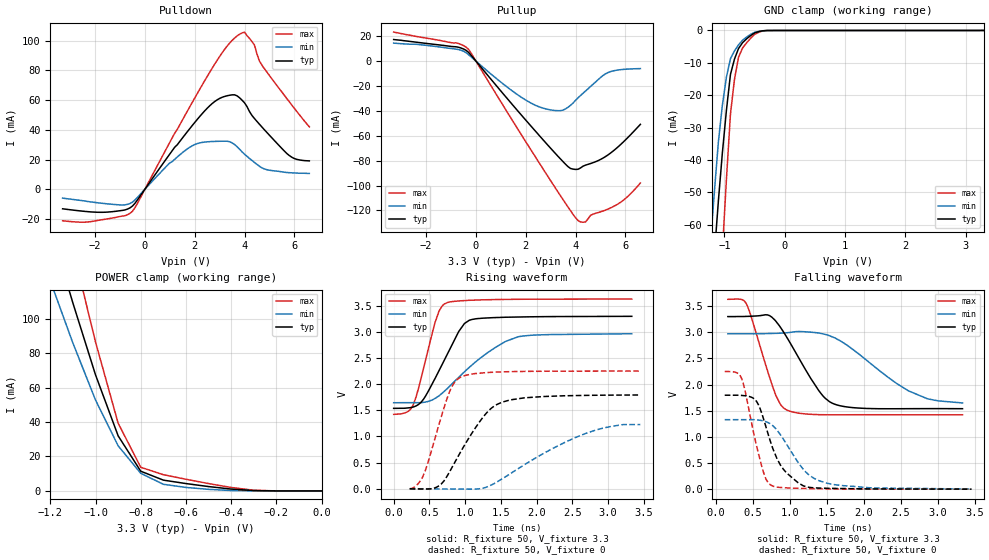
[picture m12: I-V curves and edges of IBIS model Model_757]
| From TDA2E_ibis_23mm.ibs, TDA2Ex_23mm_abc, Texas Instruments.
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| Model based on original model for BC1833DV40DCPBFBP1811_SSCEV
|   Sub model BC40D_V_10P_SC1_3P3
[model]   Model_757
|[Description]  [3.3V-I/O-X-40C CLASS MODE SLOW MODE, IND, 10 PERCENT%]
|   40C CLASS MODE SLOW MODE, ,IND,10 PERCENT%
|[Input Load]
|[Output Drive] 40C CLASS MODE SLOW MODE
|Voltage   3.3V
|Mode   I/O
Model_type   I/O
Polarity   Non-Inverting
Enable   Active-Low
Vinl =  0.8V
Vinh =  2V
Cref =  15pF
Rref =  100.0000M
Vref =  0V
Vmeas =  1.65
C_comp   2.155p   1.84p   2.47p
[Model Spec]
Vinl   0.8V   0.8V   0.8V
Vinh   2V   2V   2V
D_overshoot_ampl_h 0.66 0.66 0.66
D_overshoot_ampl_l 0.66 0.66 0.66
D_overshoot_area_h 0.33n 0.33n 0.33n
D_overshoot_area_l 0.33n 0.33n 0.33n
D_overshoot_high 3.96 3.96 3.96
D_overshoot_low -0.66 -0.66 -0.66
D_overshoot_time 1n 1n 1n
S_overshoot_high 3.3 3.3 3.3
S_overshoot_low 0 0 0
[Temperature Range]   25   125   -40
[Voltage Range]   3.3   2.97   3.63
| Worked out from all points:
|   slope of the pulldown table from 0 to 0.495 V, typ, clamps not added: 41.8 ohm
|   slope of the pullup table from 0 to 0.495 V, typ, clamps not added: 41.4 ohm
|   GND clamp passes 1 mA (typ) near -0.52 V on its own axis
|   POWER clamp passes 1 mA (typ) near -0.39 V on its own axis
|   rising waveform, R_fixture 50, V_fixture 3.3: 20-80 % time 393ps typ, 678ps min, 244ps max; typ from 1.54 V to 3.3 V
|   rising waveform, R_fixture 50, V_fixture 0: 20-80 % time 493ps typ, 965ps min, 299ps max; typ from -0.001 V to 1.79 V
|   falling waveform, R_fixture 50, V_fixture 3.3: 20-80 % time 448ps typ, 747ps min, 291ps max; typ from 3.3 V to 1.54 V
|   falling waveform, R_fixture 50, V_fixture 0: 20-80 % time 302ps typ, 402ps min, 211ps max; typ from 1.8 V to 0.001 V
[POWER_clamp]
-3.3V     1.165A     1.155A     1.459A
-1.2V     153.4mA    122mA      196.7mA
-1.167V   138.6mA    109.9mA    177.9mA
-1.1V     109.1mA    85.82mA    140.3mA
-1.067V   95.17mA    74.8mA     122.3mA
-1.033V   81.28mA    63.79mA    104.4mA
-900mV    31.99mA    26.19mA    39.32mA
-800mV    11.44mA    10.22mA    13.73mA
-700mV    6.266mA    3.856mA    9.428mA
-600mV    4.272mA    2.023mA    6.777mA
-300mV    202.9uA    25.56uA    396.8uA
0V        3.057uA    1.011uA    8.442uA
[Pulldown]
-3.3V     -13.12mA   -5.96mA    -21.19mA
-1.6V     -15.42mA   -9.62mA    -20.15mA
-500mV    -11.32mA   -8.666mA   -14.78mA
1V        23.71mA    17.75mA    31.58mA
2V        44.93mA    30.08mA    61.37mA
3V        61.12mA    32.31mA    89.33mA
3.6V      63.57mA    30.09mA    101.8mA
3.9V      59.97mA    25.19mA    105.2mA
4.4V      47.59mA    18.06mA    96.94mA
4.7V      41.87mA    14.42mA    83.43mA
5.7V      24.04mA    11.3mA     61mA
6.6V      19.1mA     10.7mA     42mA
[Pullup]
-3.3V     17.3mA     14.4mA     23.3mA
-300mV    7.112mA    5.275mA    9.555mA
1.4V      -33.47mA   -23.08mA   -45.6mA
2.5V      -58.82mA   -36.46mA   -80.5mA
3.4V      -78.75mA   -39.82mA   -108.4mA
3.8V      -86.3mA    -35.51mA   -120.3mA
4.1V      -86.92mA   -29.52mA   -128.1mA
4.4V      -83.61mA   -24.04mA   -129.3mA
4.6V      -82.33mA   -20.44mA   -124mA
5.3V      -75.41mA   -9.24mA    -118.9mA
5.9V      -65.3mA    -6.71mA    -112.1mA
6.6V      -50.83mA   -6.04mA    -97.96mA
[GND_clamp]
-3.3V     -675.1mA   -811.6mA   -985.9mA
-1.233V   -86.22mA   -66.38mA   -141.8mA
-1.167V   -69.2mA    -49.86mA   -116.5mA
-1.1V     -52.6mA    -34.38mA   -91.45mA
-1.033V   -37.65mA   -22.94mA   -67.83mA
-966.7mV  -24.63mA   -14.38mA   -45.95mA
-900mV    -13.56mA   -8.681mA   -25.81mA
-833.3mV  -8.843mA   -6.325mA   -15.09mA
-766.7mV  -5.582mA   -4.435mA   -8.297mA
-700mV    -3.779mA   -3.011mA   -5.442mA
-500mV    -752.8uA   -575uA     -1.188mA
3.3V      3.057uA    52.54uA    8.238uA
[Ramp]
dV/dt_f   1.07844/0.45734786n   0.8256/0.77814953n   1.32798/0.29199949n
dV/dt_r  1.0823181/0.49617358n  0.8034027/1.0980344n  1.3549771/0.29999862n
R_load = 50
[Rising Waveform]
R_fixture = 50
V_fixture = 3.3
V_fixture_min = 2.97
V_fixture_max = 3.63
0s        1.537V     1.645V     1.422V
182.4ps   1.543V     1.645V     1.464V
264.2ps   1.56V      1.645V     1.58V
406.5ps   1.691V     1.65V      2.235V
580.3ps   2.112V     1.728V     3.185V
710.4ps   2.463V     1.865V     3.534V
911.2ps   3.008V     2.132V     3.592V
1.101ns   3.24V      2.373V     3.607V
1.743ns   3.286V     2.907V     3.624V
3.333ns   3.298V     2.965V     3.628V
[Rising Waveform]
R_fixture = 50
V_fixture = 0
V_fixture_min = 0
V_fixture_max = 0
224.9ps   -546.1uV   -881.9uV   -364.7uV
405.5ps   -6.218mV   -881.9uV   223.7mV
639.7ps   60.19mV    -5.23mV    1.251V
807.5ps   383.3mV    -5.466mV   1.933V
938.3ps   706.7mV    -7.163mV   2.137V
1.276ns   1.411V     19.68mV    2.219V
1.523ns   1.658V     192.6mV    2.236V
2.618ns   1.784V     1.02V      2.25V
3.05ns    1.79V      1.193V     2.25V
3.453ns   1.793V     1.227V     2.251V
[Falling Waveform]
R_fixture = 50
V_fixture = 3.3
V_fixture_min = 2.97
V_fixture_max = 3.63
162.8ps   3.3V       2.97V      3.63V
409.4ps   3.303V     2.97V      3.555V
701ps     3.332V     2.976V     2.252V
812.2ps   3.21V      2.98V      1.789V
962.7ps   2.896V     2.991V     1.512V
1.392ns   1.884V     2.986V     1.425V
1.588ns   1.635V     2.904V     1.422V
2.602ns   1.539V     1.88V      1.423V
2.858ns   1.54V      1.729V     1.422V
3.333ns   1.539V     1.649V     1.423V
[Falling Waveform]
R_fixture = 50
V_fixture = 0
V_fixture_min = 0
V_fixture_max = 0
120.1ps   1.797V     1.329V     2.251V
343ps     1.793V     1.329V     2.137V
550.6ps   1.679V     1.326V     828.9mV
679ps     1.184V     1.289V     189.7mV
776.2ps   755.7mV    1.205V     55.84mV
916.5ps   375.1mV    948.3mV    28.54mV
1.114ns   121.8mV    508.9mV    17.53mV
1.281ns   32.12mV    249.4mV    9.95mV
1.503ns   17.6mV     113.8mV    6.217mV
3.453ns   844.2uV    2.89mV     609.4uV
